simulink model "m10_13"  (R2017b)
settings: Solver=VariableStepAuto  StartTime=0.0  StopTime=10.0  RelTol=1e-3

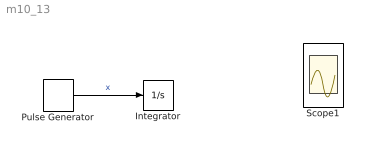
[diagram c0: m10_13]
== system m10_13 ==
  Integrator : Integrator
  Pulse Generator : DiscretePulseGenerator  PulseType=Time based  Period=10  PulseWidth=5
  Scope1 : Scope  NumInputPorts=2
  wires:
  Pulse Generator/1 -> Integrator/1  "x"
